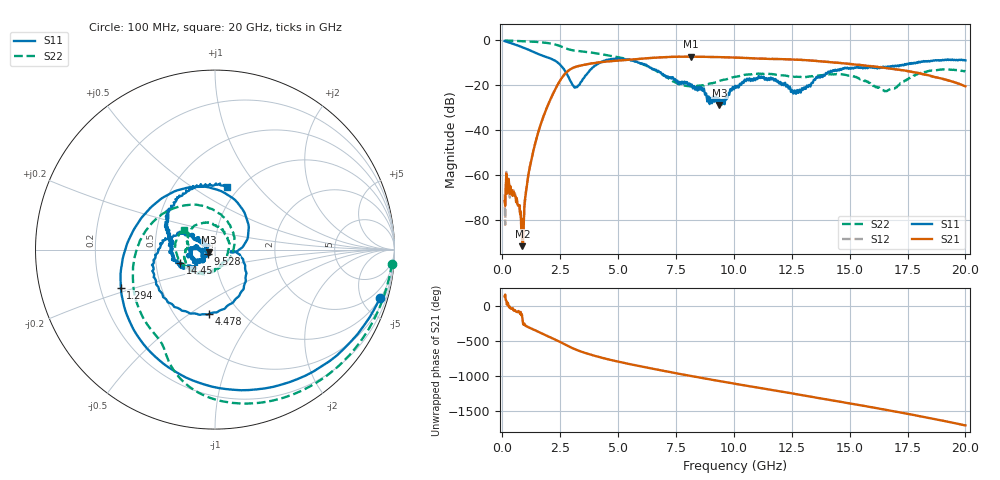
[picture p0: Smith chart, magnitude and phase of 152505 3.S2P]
!  2-Port S-parameters saved by WinCal
! VAR MeasName=S-Parameters (CALIBRATED_DATA) read from VNA (N5230C)
! VAR MeasDate=4/10/2015 9:28:44 AM
! VAR NAME=152505 3
! VAR FILENAME=152505 3.S2P
! VAR DATE=4/10/2015 9:28:44 AM
! VAR PHYS_PORTS=1,2
# Hz S DB R 50
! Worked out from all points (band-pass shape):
!   801 points, 100 MHz to 20 GHz, reference 50 ohm
!   highest |S21| = -7.31 dB at 8.159 GHz (marker M1); lowest = -91.8 dB at 871.1 MHz (marker M2)
!   |S21| within 3 dB of the highest: 3.867 GHz to 14.77 GHz (10.9 GHz wide, 117 % of centre)
!   lowest |S11| = -28.8 dB at 9.378 GHz (marker M3), VSWR 1.07, Z = 46.8 - j1.38 ohm
!   |S11| at or under -10 dB: 2.4 GHz to 4.232 GHz (1.832 GHz wide, 55.2 % of centre); 5.866622 GHz to 5.888075 GHz (21.45 MHz wide, 0.365 % of centre); 5.901 GHz to 17.87 GHz (11.97 GHz wide, 101 % of centre)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
!   |S22| runs from -22.7 to -0.1 dB; largest |S21 - S12| = 0.0071
!   S11 on the Smith chart (normalised r, x): 100 MHz: 1.03, -6.80; 1.294 GHz: 0.29, -0.18; 4.478 GHz: 0.72, -0.60; 9.528 GHz: 0.92, -0.04; 14.45 GHz: 0.67, -0.11; 20 GHz: 0.88, +0.70
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1e8  -0.37 -16.4  -71.68 141.0  -68.74 130.7  -0.08 -4.6
2.74125e8  -0.92 -41.0  -61.78 -2.5  -62.15 -2.6  -0.17 -11.5
8.71125e8  -3.12 -114.0  -91.81 -177.9  -87.02 173.3  -0.40 -35.3
1.294e9  -4.94 -157.9  -51.50 34.3  -51.58 35.1  -0.61 -52.5
1.74175e9  -6.90 160.0  -35.00 -34.4  -34.97 -34.3  -0.97 -71.4
2.3885e9  -9.89 80.4  -19.87 -133.2  -19.89 -133.2  -2.19 -100.7
3.109875e9  -20.98 -8.8  -12.04 109.7  -12.07 109.7  -4.58 -121.7
3.43325e9  -18.21 -7.8  -11.15 68.6  -11.14 68.9  -4.94 -130.6
4.478e9  -8.83 -95.6  -9.50 -31.2  -9.48 -31.0  -6.54 -166.2
5.497875e9  -8.65 -161.1  -8.66 -106.4  -8.61 -106.6  -8.70 151.3
6.741625e9  -13.63 153.0  -7.66 171.6  -7.65 171.2  -14.21 78.8
8.1595e9  -19.79 148.1  -7.31 83.0  -7.31 82.9  -20.62 -39.6
9.378375e9  -28.84 -155.9  -7.51 11.1  -7.54 11.1  -18.18 -95.8
9.527625e9  -26.38 -149.5  -7.55 2.5  -7.55 2.5  -17.66 -100.4
1.005e10  -20.35 -138.3  -7.70 -27.5  -7.72 -27.6  -16.32 -116.1
1.146788e10  -17.27 179.9  -8.27 -106.5  -8.21 -106.5  -14.98 -162.2
1.258725e10  -23.64 176.7  -8.63 -169.7  -8.62 -169.3  -16.27 175.5
1.338325e10  -18.96 -138.6  -9.10 144.7  -9.03 145.0  -16.01 166.7
1.445288e10  -13.58 -158.5  -10.00 83.5  -9.97 83.5  -15.01 135.2
1.669162e10  -11.97 167.9  -12.52 -46.9  -12.59 -48.2  -22.06 -32.1
1.835825e10  -9.49 136.3  -15.47 -151.8  -15.65 -152.0  -13.79 -158.8
2e10  -8.98 79.1  -20.52 97.1  -20.56 97.5  -13.85 147.3
